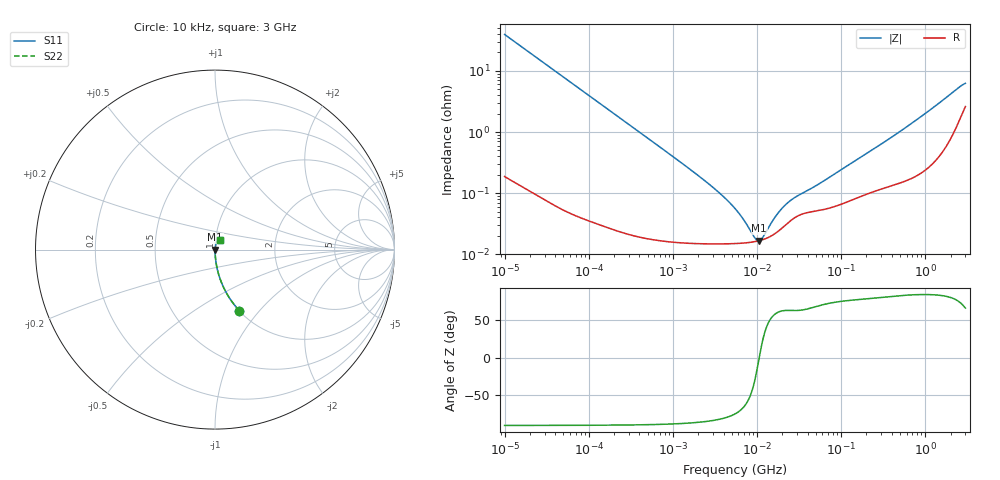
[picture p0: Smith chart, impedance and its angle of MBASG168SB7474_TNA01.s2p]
! MBASG168SB7474_TNA01  S-PARAMETER MODEL  ( Standard Model )
! Model Generated by TAIYO YUDEN Corporation (http://www.ty-top.com)
! Version 3.0
! TAIYO YUDEN Control No. 240510
! Copyright(c) 2012 TAIYO YUDEN CO.,LTD. All Rights Reserved.
! Product Description (link to TY-COMPAS)
! https://ds.yuden.co.jp/TYCOMPAS/or/detail?pn=MBASG168SB7474KTNA01&u=M
! Products Name : Multilayer Ceramic Capacitors
! Characteristics :
!  Capacitance : 0.47 [uF] , Rated Voltage : 35 [V] , TCC : X7R
!  Case Size : 1.6 x 0.8 / 0.063 x 0.031 [mm/inch] , Thickness : 0.8 / 0.031 [mm/inch]
!  (Conditions: Temperature = 25 [degC] , DC Bias Voltage = 0 [V])
! External Node Assignments :
!  1  o---| |---o  2
! GND o---------o GND
! Frequency Range : 10kHz  -  3GHz  [ 401 STEP ]
# MHZ S RI R 50
! Freq[MHz].  S11 Real  S11 Imag  S21 Real  S21 Imag  S12 Real  S12 Imag  S22 Real  S22 Imag
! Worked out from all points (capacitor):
!   401 points, 10 kHz to 3 GHz, reference 50 ohm
!   read as one part in series: C = 403 nF near 10.65 kHz
!   lowest |Z| = 16.7 mohm at 10.62 MHz (marker M1)
!   series resonance near 10.63 MHz, so ESL is about 560 pH
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0.01  0.1357 -0.3401  0.8643 0.3401  0.8643 0.3401  0.1357 -0.3401
0.016047  0.0581 -0.2314  0.9419 0.2314  0.9419 0.2314  0.0581 -0.2314
0.027426  0.0212 -0.141  0.9788 0.141  0.9788 0.141  0.0212 -0.141
0.045421  0.0081 -0.0864  0.9919 0.0864  0.9919 0.0864  0.0081 -0.0864
0.082683  0.00268 -0.0478  0.9973 0.0478  0.9973 0.0478  0.00268 -0.0478
0.683653  0.000201 -0.00582  0.9998 0.00582  0.9998 0.00582  0.000201 -0.00582
2.737278  0.000149 -0.00137  0.9999 0.00137  0.9999 0.00137  0.000149 -0.00137
3.996065  0.000148 -0.000864  0.9999 0.000864  0.9999 0.000864  0.000148 -0.000864
5.477226  0.00015 -0.00054  0.9999 0.00054  0.9999 0.00054  0.00015 -0.00054
6.829836  0.000152 -0.000347  0.9998 0.000347  0.9998 0.000347  0.000152 -0.000347
9.361346  0.00016 -9.75e-05  0.9998 9.75e-05  0.9998 9.75e-05  0.00016 -9.75e-05
9.97066  0.000163 -4.92e-05  0.9998 4.92e-05  0.9998 4.92e-05  0.000163 -4.92e-05
10.61963  0.000167 -9.11e-07  0.9998 9.11e-07  0.9998 9.11e-07  0.000167 -9.11e-07
11.67315  0.000173 7.17e-05  0.9998 -7.17e-05  0.9998 -7.17e-05  0.000173 7.17e-05
16.51234  0.000219 0.000347  0.9998 -0.000347  0.9998 -0.000347  0.000219 0.000347
21.24962  0.000291 0.000549  0.9997 -0.000549  0.9997 -0.000549  0.000291 0.000549
28.22191  0.000398 0.000751  0.9996 -0.000751  0.9996 -0.000751  0.000398 0.000751
45.28751  0.000498 0.00111  0.9995 -0.00111  0.9995 -0.00111  0.000498 0.00111
374.4521  0.00134 0.00765  0.9987 -0.00765  0.9987 -0.00765  0.00134 0.00765
964.2293  0.00265 0.0191  0.9974 -0.0191  0.9974 -0.0191  0.00265 0.0191
2482.93  0.0166 0.0494  0.9834 -0.0494  0.9834 -0.0494  0.0166 0.0494
3000  0.0284 0.0538  0.9716 -0.0538  0.9716 -0.0538  0.0284 0.0538
